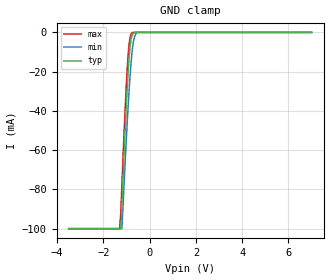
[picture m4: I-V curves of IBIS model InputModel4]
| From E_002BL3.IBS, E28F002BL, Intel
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|*********************Input Model 4*********************************
[Model]   InputModel4
Model_type   Input
|   Model for OE# pin.
Vinl = 0.8V
Vinh = 2.0V
|Variable   Typ   Min   Max
C_comp   5.61p   NA   7.6p
[Voltage Range]   3.3V   3.0V   3.6V
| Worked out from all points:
|   GND clamp passes 1 mA (typ) near -0.74 V on its own axis
[GND_clamp]
|Voltage  I(typ)   I(min)   I(max)
-3.5V     -100mA     -100mA     -100mA
-1.3V     -100mA     -100mA     -100mA
-1.25V    -100mA     -100mA     -92.37mA
-1.2V     -87.67mA   -100mA     -77.67mA
-1.05V    -47.16mA   -64.24mA   -36.63mA
-950mV    -23.96mA   -41.85mA   -14.59mA
-900mV    -14.63mA   -31.74mA   -6.958mA
-850mV    -7.671mA   -22.78mA   -2.615mA
-750mV    -1.189mA   -8.794mA   0A
-650mV    0A         -2.153mA   0A
-550mV    0A         0A         0A
7V        0A         0A         0A
[Power_clamp]
| Input buffer circuits of this product do not intrinsically
| require a [Power_clamp] definition.  This zero current
| [Power_clamp] table is provided for the compatibility with
| some IBIS parsers.
|Voltage  I(typ)   I(min)   I(max)
-3.3V     0A         0A         0A
0V        0A         0A         0A
3.3V      0A         0A         0A
7V        0A         0A         0A
